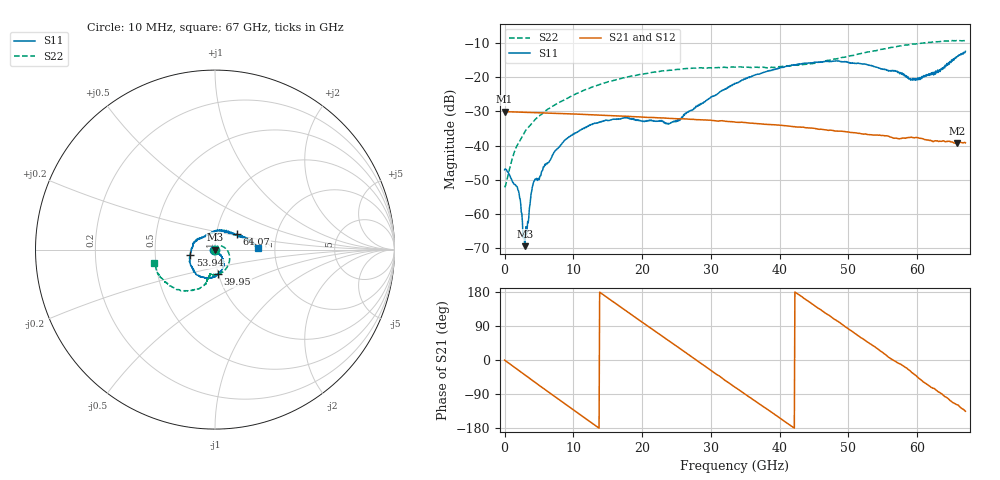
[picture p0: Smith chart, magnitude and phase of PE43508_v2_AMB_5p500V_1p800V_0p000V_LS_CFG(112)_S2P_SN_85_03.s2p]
!Keysight Technologies,N5227A,US51270237,A.10.43.00
!Date: Wednesday, August 22, 2018 17:18:23
!Correction: S11(Full 2 Port(1,3))
!S31(Full 2 Port(1,3))
!S13(Full 2 Port(1,3))
!S33(Full 2 Port(1,3))
!S2P File: Measurements: S11, S31, S13, S33:
# Hz S  dB  R 50
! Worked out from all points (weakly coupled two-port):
!   801 points, 10 MHz to 67 GHz, reference 50 ohm
!   highest |S21| = -30.04 dB at 10 MHz (marker M1); lowest = -39.3 dB at 65.74 GHz (marker M2)
!   lowest |S11| = -69.5 dB at 2.941 GHz (marker M3), VSWR 1.00, Z = 50 + j0.0306 ohm
!   |S11| at or under -10 dB: start of sweep to end of sweep
!   |S22| runs from -52.3 to -9.2 dB; largest |S21 - S12| = 0.0002
!   S11 on the Smith chart (normalised r, x): 10 MHz: 0.99, -0.00; 39.95 GHz: 1.00, -0.28; 53.94 GHz: 0.76, -0.05; 64.07 GHz: 1.26, +0.22; 67 GHz: 1.63, +0.03
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1e7  -47.12 -175.7  -30.04 -0.3  -30.04 -0.2  -52.26 -177.3
1.935962e9  -52.89 158.7  -30.18 -26.2  -30.18 -26.2  -39.58 80.3
2.270912e9  -55.74 166.1  -30.20 -30.6  -30.20 -30.6  -38.47 74.9
2.6896e9  -67.01 147.4  -30.23 -36.1  -30.23 -36.2  -36.88 68.4
2.940812e9  -69.51 66.3  -30.24 -39.5  -30.25 -39.5  -36.00 65.7
3.192025e9  -65.94 29.6  -30.26 -42.8  -30.26 -42.8  -35.29 63.5
3.945662e9  -53.39 -28.2  -30.31 -52.6  -30.31 -52.7  -33.57 55.7
4.36435e9  -50.26 -16.5  -30.34 -58.1  -30.34 -58.1  -32.57 52.3
8.634962e9  -38.71 -57.8  -30.63 -113.8  -30.63 -113.8  -26.66 21.4
1.123082e10  -35.15 -66.9  -30.83 -147.4  -30.84 -147.4  -24.08 2.5
1.74274e10  -31.89 -88.0  -31.38 132.9  -31.37 132.9  -20.08 -34.6
2.236791e10  -32.76 -83.1  -31.87 69.7  -31.87 69.6  -18.32 -59.2
2.513125e10  -32.47 -64.8  -32.15 34.8  -32.14 34.7  -17.63 -70.5
3.3505e10  -21.86 -55.5  -33.10 -71.9  -33.11 -72.0  -16.98 -95.6
3.995279e10  -17.19 -82.8  -34.01 -152.4  -34.01 -152.4  -16.83 -102.4
4.472582e10  -15.72 -106.9  -34.89 147.9  -34.87 148.0  -15.98 -102.5
5.393695e10  -16.99 -167.5  -36.91 33.4  -36.87 33.3  -12.22 -115.7
5.586291e10  -18.18 171.3  -37.32 6.8  -37.32 6.3  -11.35 -121.9
5.979858e10  -20.35 113.1  -37.65 -40.7  -37.68 -41.2  -10.21 -135.5
6.406919e10  -16.43 35.0  -38.89 -97.3  -38.96 -97.6  -9.38 -154.0
6.574394e10  -14.09 13.7  -39.33 -117.9  -39.40 -118.0  -9.23 -160.8
6.7e10  -12.37 1.8  -39.21 -135.2  -39.26 -135.4  -9.18 -167.3
